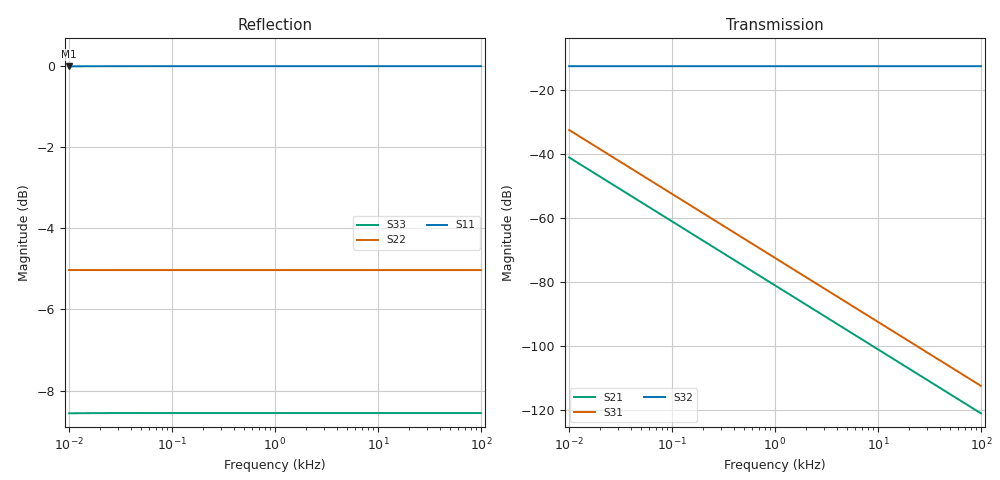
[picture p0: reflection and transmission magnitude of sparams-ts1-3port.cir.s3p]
# Hz S RI R 50 50 100
!  Freq  ReS11  ImS11  ReS12  ImS12  ReS13  ImS13
!  ReS21  ImS21  ReS22  ImS22  ReS23  ImS23
!  ReS31  ImS31  ReS32  ImS32  ReS33  ImS33
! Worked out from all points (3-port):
!   41 points, 10 Hz to 100 kHz, reference 50 ohm
!   strongest paths, dB at 10 Hz, 100 Hz, 1 kHz, 10 kHz, 100 kHz:
!     S32: -12.6, -12.6, -12.6, -12.6, -12.6
!     S31: -32.6, -52.6, -72.6, -92.6, -112.6
!     S21: -41.2, -61.2, -81.2, -101.2, -121.2
!   lowest |S11| = 0.0 dB at 10 Hz (marker M1)
!   |S11| at or under -10 dB: nowhere
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10  -0.9964 -0.0635  0.000388 -0.00872  0.00104 -0.0234
    0.000388 -0.00872  0.5605 -0.0012  0.2333 -0.00322
    0.00104 -0.0234  0.2333 -0.00322  -0.3732 -0.00866
19.95262  -0.9985 -0.0319  9.77e-05 -0.00438  0.000262 -0.0118
          9.77e-05 -0.00438  0.5605 -0.000602  0.2331 -0.00162
          0.000262 -0.0118  0.2331 -0.00162  -0.3735 -0.00434
39.81072  -0.999 -0.016  2.45e-05 -0.0022  6.59e-05 -0.0059
          2.45e-05 -0.0022  0.5604 -0.000302  0.2331 -0.000811
          6.59e-05 -0.0059  0.2331 -0.000811  -0.3736 -0.00218
125.8925  -0.9992 -0.00505  2.45e-06 -0.000694  6.59e-06 -0.00187
          2.45e-06 -0.000694  0.5604 -9.56e-05  0.2331 -0.000256
          6.59e-06 -0.00187  0.2331 -0.000256  -0.3736 -0.000689
794.3282  -0.9992 -0.000801  6.14e-08 -0.00011  1.65e-07 -0.000296
          6.14e-08 -0.00011  0.5604 -1.62e-05  0.2331 -4.11e-05
          1.65e-07 -0.000296  0.2331 -4.11e-05  -0.3736 -0.00011
1000  -0.9992 -0.000636  3.87e-08 -8.74e-05  1.04e-07 -0.000235
      3.87e-08 -8.74e-05  0.5604 -1.34e-05  0.2331 -3.29e-05
      1.04e-07 -0.000235  0.2331 -3.29e-05  -0.3736 -8.73e-05
1258.925  -0.9992 -0.000505  2.43e-08 -6.94e-05  6.57e-08 -0.000187
          2.43e-08 -6.94e-05  0.5604 -1.13e-05  0.2331 -2.64e-05
          6.57e-08 -0.000187  0.2331 -2.64e-05  -0.3736 -6.96e-05
1995.262  -0.9992 -0.000319  9.55e-09 -4.38e-05  2.6e-08 -0.000118
          9.55e-09 -4.38e-05  0.5604 -8.76e-06  0.2331 -1.73e-05
          2.6e-08 -0.000118  0.2331 -1.73e-05  -0.3736 -4.46e-05
2511.886  -0.9992 -0.000253  5.94e-09 -3.48e-05  1.63e-08 -9.35e-05
          5.94e-09 -3.48e-05  0.5604 -8.24e-06  0.2331 -1.43e-05
          1.63e-08 -9.35e-05  0.2331 -1.43e-05  -0.3736 -3.6e-05
100000  -0.9992 -6.36e-06  -2.17e-10 -8.74e-07  -2.13e-10 -2.35e-06
        -2.17e-10 -8.74e-07  0.5604 -0.000138  0.2331 -5.82e-05
        -2.13e-10 -2.35e-06  0.2331 -5.82e-05  -0.3736 -5.78e-05
